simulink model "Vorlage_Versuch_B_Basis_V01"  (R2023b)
settings: Solver=FixedStepAuto  StartTime=0.0  StopTime=inf  FixedStep=1e-3  RelTol=1e-3
undefined symbols (not defined in the file): bin2dec
libraries: simulink x9, instrumentseriallib x3, eeGeneralControl x1

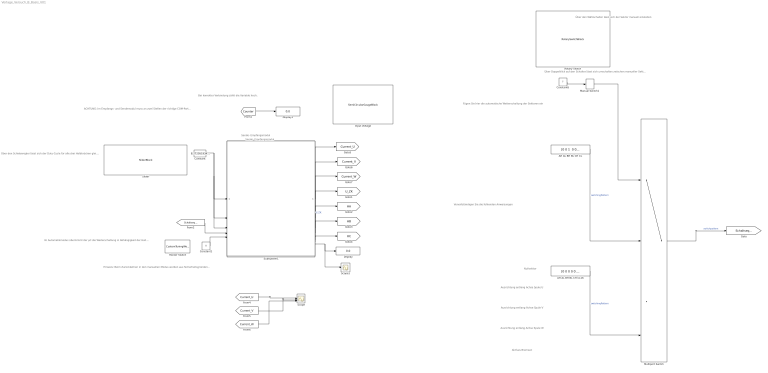
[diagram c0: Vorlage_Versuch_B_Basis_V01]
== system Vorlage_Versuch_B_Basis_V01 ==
  note: Ausrichtung entlang Achse Spule V
  note: Nullvektor
  note: Ausrichtung entlang Achse Spule U
  note: Ausrichtung entlang Achse Spule W
  note: Sende- Empfangsmodul
  note: Bei korrekter Verbindung zählt die Variable hoch.
  note: Aktives Bremsen
  note: ACHTUNG: Im Empfangs- und Sendemodul muss an zwei Stellen der richtige COM-Port ausgewählt werden. (Verfügbare Schnittstellen, siehe Windows-Systemsteuerung)
  note: Hinweis: Beim Zurückkehren in den manuellen Modus werden aus Sicherheitsgründen alle Halbbrücken deaktiviert. Erst eine Sektoränderung reaktiviert die Halbbrücken.
  note: Sende- Empfangsmodul
  note: Fügen Sie hier die automatische Weiterschaltung der Sektoren ein
  note: Über den Wählschalter lässt sich der Sektor manuell einstellen
  note: Über Doppelklick auf den Schalter lässt sich umschalten zwischen manueller Sektorwahl und automatischer Weiterschaltung
  note: Vervollständigen Sie die fehlenden Anweisungen
  note: Im Automatikmodus übernimmt der µC die Weiterschaltung in Abhängigkeit der Hall-Informationen
  note: Über den Schieberegler lässt sich der Duty-Cycle für alle drei Halbbrücken gleichzeitig einstellen.
  AH AL BH BL CH CL : Constant  Value="[0 0 1  0 0 1]"  SampleTime=-1
  AH AL BH BL CH CL16 : Constant  Value=[0 0 0 0 0 0]  SampleTime=-1
  Constant : Constant  Value=8.772051934145363
  Constant1 : Constant  Value=0
  Constant6 : Constant  Value=7  OutDataTypeStr=uint8
  Display : Display
  Display1 : Display
  Input Voltage : SemiCircularGaugeBlock  ScaleMax=25
  Manual Switch1 : ManualSwitch
  Multiport Switch : MultiPortSwitch  Inputs=11  DiagnosticForDefault=None
  Rocker Switch : CustomTuningWebBlock  LabelPosition=Hide  ShowInitialText=on  Configuration="{\"components\":[{\"name\":\"CustomSwitchStateComponent\",\"settings\":{\"position\":[0,0,1,1],\"states\":[{\"HitRegion\":{\"position\":[0,0,0.5,1]},\"Image\":{\"position\":[0.13,0,1,0.75],\"size\":[1,0.75],\"src\":\"data:image\\/svg+xml;base64,PHN2ZyB4bWxucz0iaHR0cDovL3d3dy53My5vcmcvMjAwMC9zdmciIHhtbG5zOnhsaW5rPSJodHRwOi8vd3d3LnczLm9yZy8xOTk5L3hsaW5rIiB2aWV3Qm94PSIwIDAgNzUgMjQuOCI+PGRlZnM+PHN0eWxlPi5jbHMtMXtmaWxsOnVybCgjc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"
  Rotary Switch : RotarySwitchBlock
  Scope : Scope  NumInputPorts=3
  Scope1 : Scope
  Slider : SliderBlock  TickInterval=20
  Subsystem1 : Subsystem
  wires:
  ? -> Multiport Switch/9  "switchingPattern"
  ? -> Multiport Switch/11  "switchingPattern"
  ? -> Multiport Switch/3  "switchingPattern"
  ? -> Multiport Switch/7  "switchingPattern"
  AH AL BH BL CH CL/1 -> Multiport Switch/2  "switchingPattern"
  ? -> Multiport Switch/4  "switchingPattern"
  Multiport Switch/1 -> [Schaltsequenz]  "switchpattern"
  AH AL BH BL CH CL16/1 -> Multiport Switch/8  "switchingPattern"
  ? -> Multiport Switch/5  "switchingPattern"
  ? -> Multiport Switch/10  "switchingPattern"
  Constant6/1 -> Manual Switch1/1
  Manual Switch1/1 -> Multiport Switch/1
  ? -> Multiport Switch/6  "switchingPattern"
  Subsystem1/4(U_ZK [V]) -> [U_ZK]  "U_ZK"
  [Schaltsequenz] -> Subsystem1/4(Sequence UH UL VH VL WH WL)
  Subsystem1/5(_HA) -> [HA]
  Subsystem1/6(_HB) -> [HB]
  Subsystem1/7(_HC) -> [HC]
  Subsystem1/8(" RPM [1/min]") -> Scope1/1, Display/1
  [Counter] -> Display1/1
  Constant/1 -> Subsystem1/3(Duty W [%]), Subsystem1/2(Duty V [%]), Subsystem1/1(Duty U [%])
  Constant1/1 -> Subsystem1/5(BLDC Auto)
  ? -> Multiport Switch/12  "switchingPattern"
  Subsystem1/1(Current_U) -> [Current_U]
  Subsystem1/2(Current_V) -> [Current_V]
  Subsystem1/3(Current_W) -> [Current_W]
  [Current_U] -> Scope/1
  [Current_V] -> Scope/2
  [Current_W] -> Scope/3

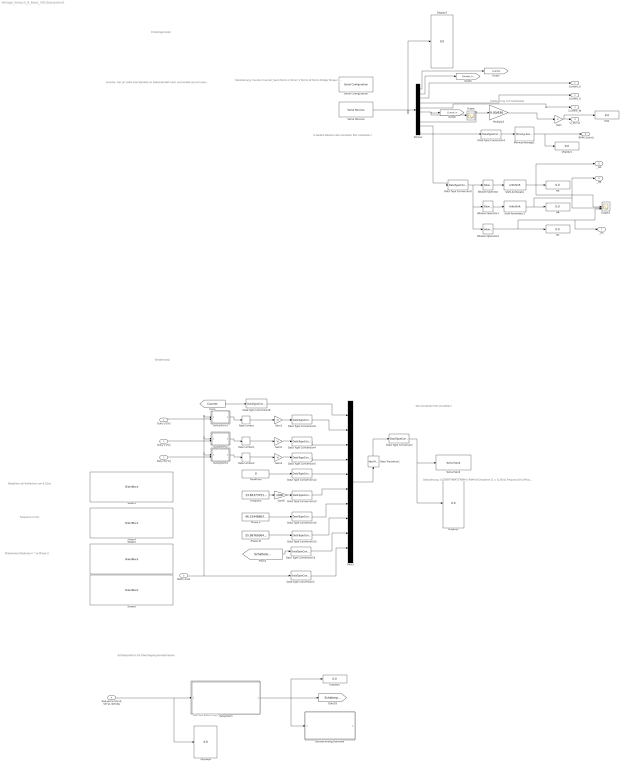
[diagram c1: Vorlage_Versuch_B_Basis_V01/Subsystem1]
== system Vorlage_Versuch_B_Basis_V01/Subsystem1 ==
  note: Counter: Der µC zählt eine Variable im Sekundentakt hoch und sendet sie zum Host Counter_Send: Der empfangene Wert wird wieder nach unten gesendet und sofort wieder empfangen Die Variable läuft ein mal im Kreis. Zählen beide Werte hoch ist alles in Ordnung. Zählt nur der Counter hoch bedeutet das, dass der Ursprungscounter nicht zurückgesendet wurde bzw. allgemein kein Daten von Simulink zum µC übertragen werden.
  note: Dekodierung: Counter Counter_Send Strom U Strom V Strom W Strom Bridge Torque U Zwischenkreis Hall Drehzahl
  note: Kalibrierung mit Oszilloskop
  note: Dekodierung: Counter PWM U PWM V PWM W Deadtime [1 = 6,25ns] Frequenz [Hz] Phase V PHase W Schaltsequenz BLDC Automatic
  note: Deadtime als Vielfaches von 6,25ns
  note: Frequenz in kHz
  note: Phasenverschiebung in ° zu Phase U
  note: Den korrekten Port einstellen!
  note: Sendemodul
  note: Empfangsmodul
  note: In beiden Blöcken den korrekten Port einstelllen!
  note: Schalterpattern für Übertragung komplrimieren
  note: Gibt das Pattern aus
  Duty U [%] : Inport
  Duty V [%] : Inport  Port=2
  Duty W [%] : Inport  Port=3
  Sequence UH UL VH VL WH WL : Inport  Port=4
  BLDC Auto : Inport  Port=5
  Bitwise Operator : simulink/Logic and Bit Operations/Bitwise Operator  logicop=AND  UseBitMask=on  BitMask=bin2dec('00000100')  BitMaskRealWorld=Stored Integer
  Bitwise Operator1 : simulink/Logic and Bit Operations/Bitwise Operator  logicop=AND  UseBitMask=on  BitMask=bin2dec('00000010')  BitMaskRealWorld=Stored Integer
  Bitwise Operator2 : simulink/Logic and Bit Operations/Bitwise Operator  logicop=AND  UseBitMask=on  BitMask=bin2dec('00000001')  BitMaskRealWorld=Stored Integer
  Data Type Conversion{,3..5,8..9,12..16} (11 alike) : DataTypeConversion  OutDataTypeStr=uint16
  Data Type Conversion1 : DataTypeConversion  OutDataTypeStr=double
  Data Type Conversion2 : DataTypeConversion  OutDataTypeStr=uint8
  Deadtime : Constant  Value=0  OutDataTypeStr=uint16
  Demux : Demux  Outputs=10
  Display{1..2,5..7} (5 alike) : Display
  Frequenz : Constant  Value=13.65373751749638  OutDataTypeStr=uint16
  Gain : Gain
  Gain1 : Gain  Gain=10
  Gain2 : Gain  Gain=10
  Gain3 : Gain  Gain=10
  Gain6 : Gain  Gain=1000
  HA : Display
  HA1 : Display
  HB : Display
  HC : Display
  Moving Average1 : eeGeneralControl/Moving Average  VariantControl=Variant1  LabelModeActiveChoice=Discrete  f=2  x0=0  BufferSize=8192  Ts=-1
  Multiply1 : Gain  Gain=9.00/836
  Mux2 : Mux  Inputs=10
  Phase V : Constant  Value=46.15448863811867  OutDataTypeStr=uint16
  Phase W : Constant  Value=55.99769364620121  OutDataTypeStr=uint16
  Rate Limiter : RateLimiter  RisingSlewLimit=200  FallingSlewLimit=-200
  Rate Limiter1 : RateLimiter  RisingSlewLimit=200  FallingSlewLimit=-200
  Rate Limiter2 : RateLimiter  RisingSlewLimit=200  FallingSlewLimit=-200
  Rate Transition1 : RateTransition  OutPortSampleTime=0.05
  Rückrechnung_Kontrolle : Subsystem
  Scope : Scope
  Scope3 : Scope  NumInputPorts=3
  Serial Configuration : instrumentseriallib/Serial Configuration  Priority=-200000  PortSel=COM22  Port=COM22  ComPort=COM22  BaudRate=115000  DataBits=8  Parity=even  StopBits=1  ByteOrder=little-endian  FlowControl=none  Timeout=10  SimulateUsing=Interpreted execution  BlockInModel=on  aMode=1
  Serial Receive : instrumentseriallib/Serial Receive  Priority=1  PortSel=COM22  Port=COM22  ComPort=COM22  DataType=uint16  SaveDataType=uint8  ToggleHeader=on  Header=['X']  ToggleTerminator=on  Terminator=Custom terminator  CustomTerminator=['Y']  InputFormat=Column major  ToggleDataSize=on  DataSize=[1 10]  EnableBlockingMode=off  ActionDataUnavailable=Output last received value  ActionWhenDataUnavailable=Output last received value  CustomValue=42  SampleTime=0.001  SimulateUsing=Interpreted execution  BlockInModel=on  aMode=1
  Serial Send : instrumentseriallib/Serial Send  Priority=1  PortSel=COM22  Port=COM22  ComPort=COM22  Header=[]  Terminator=<none>  CustomTerminator=[]  EnableBlockingMode=off  SimulateUsing=Interpreted execution  BlockInModel=on  aMode=1
  Shift Arithmetic : ArithShift  BitShiftNumber=2  BitShiftDirection=Right
  Shift Arithmetic1 : ArithShift  BitShiftNumber=1  BitShiftDirection=Right
  Slider3 : SliderBlock  ScaleMax=500  TickInterval=50
  Slider4 : SliderBlock  ScaleMax=50  TickInterval=10
  Slider5 : SliderBlock  ScaleMax=180  TickInterval=20
  Slider6 : SliderBlock  ScaleMax=180  TickInterval=20
  Subsystem : Subsystem
  Subsystem1 : Subsystem
  Subsystem2 : Subsystem
  Subsystem3 : Subsystem
  Current_U : Outport
  Current_V : Outport  Port=2
  Current_W : Outport  Port=3
  U_ZK [V] : Outport  Port=4
  _HA : Outport  Port=5
  _HB : Outport  Port=6
  _HC : Outport  Port=7
  " RPM [1/min]" : Outport  Port=8
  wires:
  Demux/4 -> Current_V/1
  Data Type Conversion1/1 -> Moving Average1/1
  Serial Receive/1 -> Demux/1, Display7/1
  Demux/3 -> Current_U/1
  Moving Average1/1 -> " RPM [1/min]"/1, Display1/1
  Demux/5 -> Current_W/1
  Demux/6 -> Scope/1, [Current_In]
  Demux/2 -> [Counter_Send]
  Multiply1/1 -> Gain/1
  Demux/10 -> Data Type Conversion1/1
  Bitwise Operator1/1 -> Shift Arithmetic1/1
  Data Type Conversion2/1 -> Bitwise Operator2/1, Bitwise Operator1/1, Bitwise Operator/1
  Bitwise Operator/1 -> Shift Arithmetic/1
  Shift Arithmetic/1 -> _HA/1, Scope3/1, HA/1
  Shift Arithmetic1/1 -> _HB/1, Scope3/2, HB/1
  Bitwise Operator2/1 -> HC/1, _HC/1, Scope3/3
  Demux/8 -> Multiply1/1
  Demux/9 -> Data Type Conversion2/1
  Demux/1 -> [Counter]
  Data Type Conversion15/1 -> Mux2/8
  Phase W/1 -> Data Type Conversion15/1
  Data Type Conversion12/1 -> Mux2/5
  Gain6/1 -> Data Type Conversion13/1
  Phase V/1 -> Data Type Conversion14/1
  Data Type Conversion16/1 -> Mux2/9
  Frequenz/1 -> Gain6/1
  Data Type Conversion13/1 -> Mux2/6
  Data Type Conversion8/1 -> Mux2/1
  Deadtime/1 -> Data Type Conversion12/1
  Data Type Conversion9/1 -> Mux2/2
  Rate Transition1/1 -> Data Type Conversion/1
  Mux2/1 -> Rate Transition1/1
  Gain1/1 -> Data Type Conversion9/1
  Data Type Conversion/1 -> Display2/1, Serial Send/1
  Data Type Conversion14/1 -> Mux2/7
  Data Type Conversion3/1 -> Mux2/10
  [Counter] -> Data Type Conversion8/1
  Gain/1 -> HA1/1, U_ZK [V]/1
  Gain2/1 -> Data Type Conversion4/1
  Data Type Conversion4/1 -> Mux2/3
  Data Type Conversion5/1 -> Mux2/4
  Gain3/1 -> Data Type Conversion5/1
  BLDC Auto/1 -> Data Type Conversion3/1, Subsystem3/1(Auto), Subsystem1/1(Auto), Subsystem2/1(Auto)
  Subsystem/1(Out1) -> Rückrechnung_Kontrolle/1(In1), [Schalterpattern], Display5/1
  Sequence UH UL VH VL WH WL/1 -> Display6/1, Subsystem/1(switchpattern)
  [Schalterpattern] -> Data Type Conversion16/1
  Rate Limiter/1 -> Gain1/1
  Rate Limiter1/1 -> Gain2/1
  Rate Limiter2/1 -> Gain3/1
  Subsystem1/1(Out1) -> Rate Limiter/1
  Duty U [%]/1 -> Subsystem1/2(Duty U [%])
  Subsystem2/1(Out1) -> Rate Limiter1/1
  Duty V [%]/1 -> Subsystem2/2(Duty U [%])
  Subsystem3/1(Out1) -> Rate Limiter2/1
  Duty W [%]/1 -> Subsystem3/2(Duty U [%])

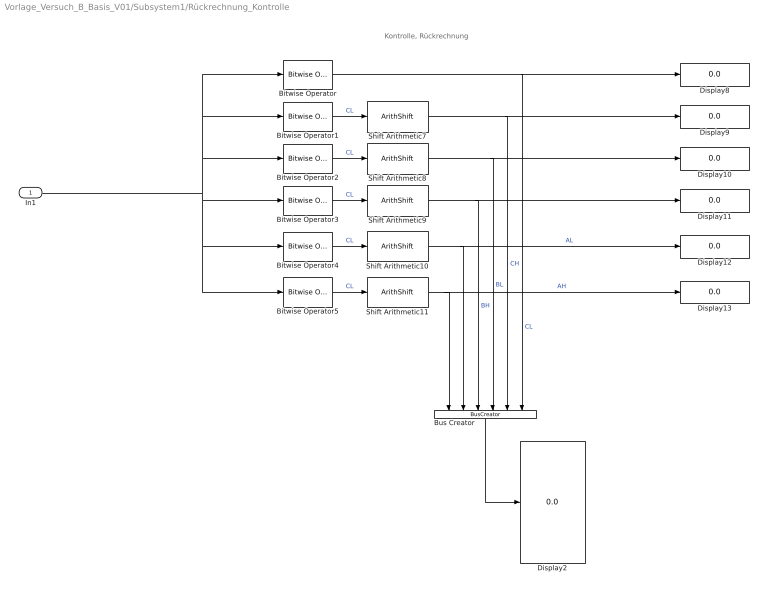
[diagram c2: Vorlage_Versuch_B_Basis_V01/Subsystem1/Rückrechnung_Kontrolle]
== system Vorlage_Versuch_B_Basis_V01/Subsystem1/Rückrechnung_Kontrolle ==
  note: Kontrolle, Rückrechnung
  In1 : Inport
  Bitwise Operator : simulink/Logic and Bit Operations/Bitwise Operator  logicop=AND  UseBitMask=on  BitMask=0x01  BitMaskRealWorld=Stored Integer
  Bitwise Operator1 : simulink/Logic and Bit Operations/Bitwise Operator  logicop=AND  UseBitMask=on  BitMask=0x02  BitMaskRealWorld=Stored Integer
  Bitwise Operator2 : simulink/Logic and Bit Operations/Bitwise Operator  logicop=AND  UseBitMask=on  BitMask=0x04  BitMaskRealWorld=Stored Integer
  Bitwise Operator3 : simulink/Logic and Bit Operations/Bitwise Operator  logicop=AND  UseBitMask=on  BitMask=0x08  BitMaskRealWorld=Stored Integer
  Bitwise Operator4 : simulink/Logic and Bit Operations/Bitwise Operator  logicop=AND  UseBitMask=on  BitMask=0x10  BitMaskRealWorld=Stored Integer
  Bitwise Operator5 : simulink/Logic and Bit Operations/Bitwise Operator  logicop=AND  UseBitMask=on  BitMask=0x20  BitMaskRealWorld=Stored Integer
  Bus Creator : BusCreator  Inputs=6
  Display{2,8..13} (7 alike) : Display
  Shift Arithmetic10 : ArithShift  BitShiftNumber=4  BitShiftDirection=Right
  Shift Arithmetic11 : ArithShift  BitShiftNumber=5  BitShiftDirection=Right
  Shift Arithmetic7 : ArithShift  BitShiftNumber=1  BitShiftDirection=Right
  Shift Arithmetic8 : ArithShift  BitShiftNumber=2  BitShiftDirection=Right
  Shift Arithmetic9 : ArithShift  BitShiftNumber=3  BitShiftDirection=Right
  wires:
  Shift Arithmetic8/1 -> Bus Creator/4, Display10/1  "BL"
  Shift Arithmetic9/1 -> Bus Creator/3, Display11/1  "BH"
  In1/1 -> Bitwise Operator/1, Bitwise Operator1/1, Bitwise Operator2/1, Bitwise Operator5/1, Bitwise Operator4/1, Bitwise Operator3/1
  Bitwise Operator2/1 -> Shift Arithmetic8/1  "CL"
  Shift Arithmetic7/1 -> Bus Creator/5, Display9/1  "CH"
  Shift Arithmetic10/1 -> Display12/1, Bus Creator/2  "AL"
  Bitwise Operator5/1 -> Shift Arithmetic11/1  "CL"
  Shift Arithmetic11/1 -> Display13/1, Bus Creator/1  "AH"
  Bitwise Operator/1 -> Bus Creator/6, Display8/1  "CL"
  Bus Creator/1 -> Display2/1
  Bitwise Operator1/1 -> Shift Arithmetic7/1  "CL"
  Bitwise Operator4/1 -> Shift Arithmetic10/1  "CL"
  Bitwise Operator3/1 -> Shift Arithmetic9/1  "CL"

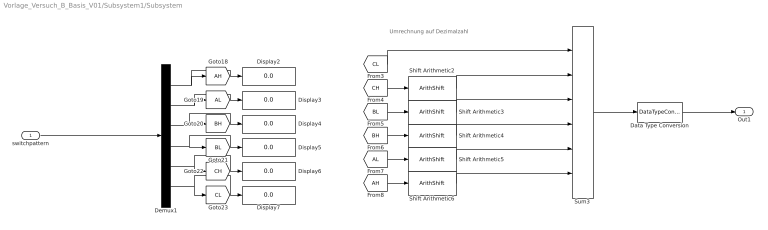
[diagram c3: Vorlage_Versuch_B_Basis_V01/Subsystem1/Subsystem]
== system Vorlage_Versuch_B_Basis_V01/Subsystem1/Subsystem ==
  note: Umrechnung auf Dezimalzahl
  switchpattern : Inport
  Data Type Conversion : DataTypeConversion  OutDataTypeStr=uint8
  Demux1 : Demux  Outputs=6
  Display{2..7} (6 alike) : Display
  Shift Arithmetic2 : ArithShift  BitShiftNumber=1  BitShiftDirection=Left
  Shift Arithmetic3 : ArithShift  BitShiftNumber=2  BitShiftDirection=Left
  Shift Arithmetic4 : ArithShift  BitShiftNumber=3  BitShiftDirection=Left
  Shift Arithmetic5 : ArithShift  BitShiftNumber=4  BitShiftDirection=Left
  Shift Arithmetic6 : ArithShift  BitShiftNumber=5  BitShiftDirection=Left
  Sum3 : Sum  Inputs=|++++++
  Out1 : Outport
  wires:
  [CL] -> Sum3/1
  Demux1/2 -> Display3/1, [AL]
  Demux1/4 -> [BL], Display5/1
  Demux1/5 -> Display6/1, [CH]
  Demux1/3 -> Display4/1, [BH]
  Shift Arithmetic4/1 -> Sum3/4
  Shift Arithmetic2/1 -> Sum3/2
  Demux1/1 -> [AH], Display2/1
  Data Type Conversion/1 -> Out1/1
  [AL] -> Shift Arithmetic5/1
  Demux1/6 -> Display7/1, [CL]
  [CH] -> Shift Arithmetic2/1
  Shift Arithmetic3/1 -> Sum3/3
  Shift Arithmetic6/1 -> Sum3/6
  [BH] -> Shift Arithmetic4/1
  [AH] -> Shift Arithmetic6/1
  Sum3/1 -> Data Type Conversion/1
  Shift Arithmetic5/1 -> Sum3/5
  [BL] -> Shift Arithmetic3/1
  switchpattern/1 -> Demux1/1

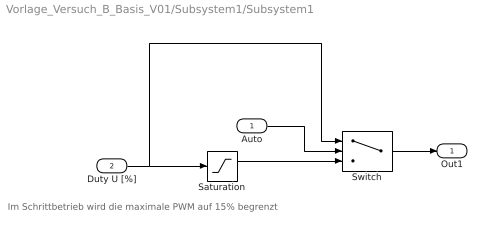
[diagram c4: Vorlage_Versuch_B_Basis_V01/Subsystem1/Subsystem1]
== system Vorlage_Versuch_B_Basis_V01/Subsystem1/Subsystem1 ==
  note: Im Schrittbetrieb wird die maximale PWM auf 15% begrenzt
  Auto : Inport
  Duty U [%] : Inport  Port=2
  Saturation : Saturate  UpperLimit=15  LowerLimit=0
  Switch : Switch  Criteria=u2 > Threshold
  Out1 : Outport
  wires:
  Saturation/1 -> Switch/3
  Auto/1 -> Switch/2
  Duty U [%]/1 -> Switch/1, Saturation/1
  Switch/1 -> Out1/1

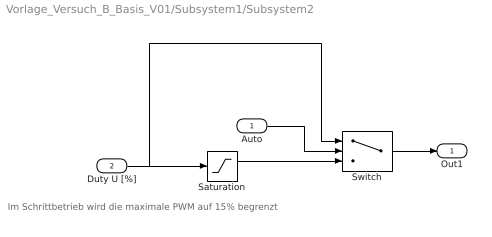
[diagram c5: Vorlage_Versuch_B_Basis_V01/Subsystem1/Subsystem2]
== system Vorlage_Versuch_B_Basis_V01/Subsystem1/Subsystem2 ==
  note: Im Schrittbetrieb wird die maximale PWM auf 15% begrenzt
  Auto : Inport
  Duty U [%] : Inport  Port=2
  Saturation : Saturate  UpperLimit=15  LowerLimit=0
  Switch : Switch  Criteria=u2 > Threshold
  Out1 : Outport
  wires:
  Saturation/1 -> Switch/3
  Auto/1 -> Switch/2
  Duty U [%]/1 -> Switch/1, Saturation/1
  Switch/1 -> Out1/1

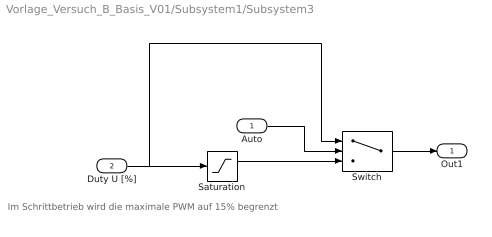
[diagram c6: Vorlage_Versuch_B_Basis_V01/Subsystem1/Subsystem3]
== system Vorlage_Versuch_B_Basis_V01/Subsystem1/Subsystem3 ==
  note: Im Schrittbetrieb wird die maximale PWM auf 15% begrenzt
  Auto : Inport
  Duty U [%] : Inport  Port=2
  Saturation : Saturate  UpperLimit=15  LowerLimit=0
  Switch : Switch  Criteria=u2 > Threshold
  Out1 : Outport
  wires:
  Saturation/1 -> Switch/3
  Auto/1 -> Switch/2
  Duty U [%]/1 -> Switch/1, Saturation/1
  Switch/1 -> Out1/1
